|   stm32f768a_778a_769_779_wlcsp180 IBIS Model
[IBIS ver]   4.2
[File name]  stm32f768a_778a_769_779_wlcsp180.ibs
[File Rev]   1.0
[Date]   24-06-2015
[Source] Data Created at STMicroelectronics
[Notes]   File originated from ELDO simulations.
[Disclaimer]  This information is for modeling purpose only and is
   not guaranted. The information is subject to change without
   notice.
[Copyright] Copyright 2016 STMicroelectronics Inc.
[Component] stm32f768a_778a_769_779_wlcsp180
[Manufacturer] STMicroelectronics
[Package]
| variable   typ   min   max
R_pkg   0.0   NA   NA
L_pkg   0.0H   NA   NA
C_pkg   0.0F   NA   NA
[Pin]   signal_name   model_name   R_pin   L_pin   C_pin
E10 PE2 io8p_arsudq_ft
F10 PE3 io8p_arsudq_ft
C12 PE4 io8p_arsudq_ft
D12 PE5 io8p_arsudq_ft
E11 PE6 io8p_arsudq_ft
C13 VBAT POWER
D13 PC13 io8p_arwsudq_ft_v33
E12 PC14-OSC32_IN io8p_arwsudq_ft_v33
E13 PC15-OSC32_OUT io8p_arsudq_ft
G10 PI9 io8p_arsudq_ft
H10 PI10 io8p_arsudq_ft
F11 PI11 io8p_arsudq_ft_v33
F13 VSS GND
F12 VDD POWER
G11 PF0 io8p_arsudq_i2cin_ft
G12 PF1 io8p_arsudq_i2cin_ft
G13 PF2 io8p_arsudq_ft
H11 PF3 io8p_arwsudq_ft
H12 PF4 io8p_arwsudq_ft
H13 PF5 io8p_arwsudq_ft
J13 VSS GND
J12 VDD POWER
K11 PF10 io8p_arwsudq_ft
K12 PH0-OSC_IN io8p_arsudq_ft
K13 PH1-OSC_OUT io8p_arsudq_ft
L11 NRST ioreset_ft_v33
L12 PC0 io8p_ar3wsudq_ft
L13 PC1 io8p_ar3wsudq_ft_v33
M11 VSSA GND
M12 VDDA POWER
M13 PA0-WKUP io8p_ar3wsudq_ft_v33
J11 PA1 io8p_ar3wsudq_ft
J10 PA2 io8p_ar3wsudq_ft_v33
L10 PH2 io8p_arsudq_ft
K10 PH3 io8p_arsudq_ft
N12 PH4 io8p_arsudq_i2cin_ft
N11 PH5 io8p_arsudq_i2cin_ft
M10 PA3 io8p_ar3wsudq_ft
J9 VSS GND
K9 VDD POWER
L9 PA4 io8p_ar3wsudq_ft
Q11 PA5 io8p_ar3wsudq_ft
N10 PA6 io8p_ar3wsudq_ft
M9 PA7 io8p_ar3wsudq_ft
P10 PB0 io8p_ar3wsudq_ft
J8 PB1 io8p_ar3wsudq_ft
J7 PB2 io8p_ar3wsudq_ft
N9 PF11 io8p_arsudq_ft
K7 PF12 io8p_arsudq_ft
Q9 VSS GND
M8 VDD POWER
L8 PF13 io8p_arsudq_ft
K8 PF14 io8p_arsudq_i2cin_ft
Q8 PF15 io8p_arsudq_i2cin_ft
N8 PG0 io8p_arsudq_ft
L7 PG1 io8p_arsudq_ft
M7 PE7 io8p_arsudq_ft
N7 PE8 io8p_arsudq_ft
P7 PE9 io8p_arsudq_ft
J6 PE10 io8p_arsudq_ft
K6 PE11 io8p_arsudq_ft
L6 PE12 io8p_arsudq_ft
P6 PE13 io8p_arsudq_ft
N6 PE14 io8p_arsudq_ft
M6 PE15 io8p_ar3wsudq_ft
K5 PB10 io8p_arsudq_i2cin_ft
L5 PB11 io8p_arsudq_i2cin_ft
P5 VCAP_1 POWER
N5 VSS GND
P4 VDD POWER
M5 PH8 io8p_arsudq_i2cin_ft
K4 PH9 io8p_arsudq_ft
L4 PH10 io8p_arsudq_ft
M4 PH11 io8p_arsudq_i2cin_ft
P3 PH12 io8p_arsudq_i2cin_ft
N4 VSS GND
H8 PB12 io8usb_id_otg_ft
J5 PB13 io8usb_vbus_otg_ft
N3 PB14 io8usb_lsfs_otg_ft
N2 PB15 io8usb_lsfs_otg_ft
M3 PD8 io8p_arsudq_ft
L3 PD9 io8p_arsudq_ft
M2 PD10 io8p_arsudq_ft
K3 PD11 io8p_arsudq_ft
J4 PD12 io8p_arsudq_i2cin_ft
L2 PD13 io8p_arsudq_i2cin_ft
M1 VSS GND
L1 PD14 io8p_arsudq_ft
K2 PD15 io8p_arsudq_ft
K1 VDDDSI POWER
H6 VCAPDSI POWER
J3 VDD12DSI POWER
J1 DSI_D0P NC
J2 DSI_D0N NC
H5 VSSDSI GND
H4 DSI_CKP NC
H3 DSI_CKN NC
H1 DSI_D1P NC
H2 DSI_D1N NC
H9 PG2 io8p_arsudq_ft
G9 PG3 io8p_arsudq_ft
G1 PG4 io8p_arsudq_ft
G2 PG5 io8p_arsudq_ft
G3 PG6 io8p_arsudq_ft
G4 PG7 io8p_arsudq_ft
G5 PG8 io8p_arsudq_ft
F1 VSS GND
F2 VDDUSB POWER
G6 PC6 io8p_arsudq_ft
F3 PC7 io8p_arsudq_ft
G8 PC8 io8p_arsudq_ft
E1 PC9 io8p_arsudq_i2cin_ft
E2 PA8 io8p_arsudq_i2cin_ft
F4 PA9 io8usb_vbus_otg_ft
F5 PA10 io8usb_id_otg_ft
E3 PA11 io8usb_lsfs_otg_ft
D1 PA12 io8usb_lsfs_otg_ft
D2 PA13 io8p_arsudq_ft
C1 VCAP_2 POWER
C2 VSS POWER
B2 VDD POWER
F6 PH13 io8p_arsudq_ft
F7 PH14 io8p_arsudq_ft
E5 PH15 io8p_arsudq_ft
E4 PI0 io8p_arsudq_ft
B3 PI1 io8p_arsudq_ft
C3 PI2 io8p_arsudq_ft
D3 PI3 io8p_arsudq_ft
A3 PA14 io8p_arsudq_ft
F8 PA15 io8p_arsudq_ft
B4 PC10 io8p_arsudq_ft
C4 PC11 io8p_arsudq_ft
D4 PC12 io8p_arsudq_ft
A4 PD0 io8p_arsudq_ft
D5 PD1 io8p_arsudq_ft
D6 PD2 io8p_arsudq_ft
B5 PD3 io8p_arsudq_ft
A5 PD4 io8p_arsudq_ft
C5 PD5 io8p_arsudq_ft
B6 VSS GND
A6 VDDSDMMC POWER
E6 PD6 io8p_arsudq_ft
E7 PD7 io8p_arsudq_ft
C6 PG9 io8p_arsudq_ft
A7 PG10 io8p_arsudq_ft
B7 PG11 io8p_arsudq_ft
D7 PG12 io8p_arsudq_ft
C7 PG13 io8p_arsudq_ft
A8 VSS GND
B8 VDD POWER
F9 PG15 io8p_arsudq_ft
E8 PB3 io8p_arsudq_ft
D8 PB4 io8p_arsudq_ft
A9 PB5 io8p_ar3wsudq_ft
B9 PB6 io8p_arsudq_i2cin_ft
C8 PB7 io8p_arsudq_i2cin_ft
A10 BOOT0 vpp_test_hv
E9 PB8 io8p_arsudq_i2cin_ft
D9 PB9 io8p_arsudq_i2cin_ft
C9 PE0 io8p_arsudq_ft
B10 PE1 io8p_arsudq_ft
A11 VSS GND
C10 PDR_ON NC
B11 VDD POWER
D10 PI4 io8p_arsudq_ft
D11 PI5 io8p_arsudq_ft
C11 PI6 io8p_arsudq_ft
B12 PI7 io8p_arsudq_ft
[Diff Pin]   inv_pin   vdiff   tdelay_typ  tdelay_min  tdelay_max
E3   D1   200mV   NA   NA   NA
N3   N2   200mV   NA   NA   NA
[Model Selector] io8p_ar3wsudq_ft
io8p00_ar3wsudq_ft_pd_lv  "SPEED00 1P8V, PD=40kOhm"
io8p00_ar3wsudq_ft_pu_lv  "SPEED00 1P8V, PU=40kOhm"
io8p00_ar3wsudq_ft_lv  "SPEED00 1P8V"
io8p01_ar3wsudq_ft_pd_lv  "SPEED01 1P8V, PD=40kOhm"
io8p01_ar3wsudq_ft_pu_lv  "SPEED01 1P8V, PU=40kOhm"
io8p01_ar3wsudq_ft_lv  "SPEED01 1P8V"
io8p10_ar3wsudq_ft_pd_lv  "SPEED10 1P8V, PD=40kOhm"
io8p10_ar3wsudq_ft_pu_lv  "SPEED10 1P8V, PU=40kOhm"
io8p10_ar3wsudq_ft_lv  "SPEED10 1P8V"
io8p11_ar3wsudq_ft_pd_lv  "SPEED11 1P8V, PD=40kOhm"
io8p11_ar3wsudq_ft_pu_lv  "SPEED11 1P8V, PU=40kOhm"
io8p11_ar3wsudq_ft_lv  "SPEED11 1P8V"
io8p00_ar3wsudq_ft_pd  "SPEED00, PD=40kOhm"
io8p00_ar3wsudq_ft_pu  "SPEED00, PU=40kOhm"
io8p00_ar3wsudq_ft  "SPEED00"
io8p01_ar3wsudq_ft_pd  "SPEED01, PD=40kOhm"
io8p01_ar3wsudq_ft_pu  "SPEED01, PU=40kOhm"
io8p01_ar3wsudq_ft  "SPEED01"
io8p10_ar3wsudq_ft_pd  "SPEED10, PD=40kOhm"
io8p10_ar3wsudq_ft_pu  "SPEED10, PU=40kOhm"
io8p10_ar3wsudq_ft  "SPEED10"
io8p11_ar3wsudq_ft_pd  "SPEED11, PD=40kOhm"
io8p11_ar3wsudq_ft_pu  "SPEED11, PU=40kOhm"
io8p11_ar3wsudq_ft  "SPEED11"
[Model Selector] io8p_ar3wsudq_ft_v33
io8p00_ar3wsudq_ft_v33_pd_lv  "SPEED00 1P8V, PD=40kOhm"
io8p00_ar3wsudq_ft_v33_pu_lv  "SPEED00 1P8V, PU=40kOhm"
io8p00_ar3wsudq_ft_v33_lv  "SPEED00 1P8V"
io8p01_ar3wsudq_ft_v33_pd_lv  "SPEED01 1P8V, PD=40kOhm"
io8p01_ar3wsudq_ft_v33_pu_lv  "SPEED01 1P8V, PU=40kOhm"
io8p01_ar3wsudq_ft_v33_lv  "SPEED01 1P8V"
io8p10_ar3wsudq_ft_v33_pd_lv  "SPEED10 1P8V, PD=40kOhm"
io8p10_ar3wsudq_ft_v33_pu_lv  "SPEED10 1P8V, PU=40kOhm"
io8p10_ar3wsudq_ft_v33_lv  "SPEED10 1P8V"
io8p11_ar3wsudq_ft_v33_pd_lv  "SPEED11 1P8V, PD=40kOhm"
io8p11_ar3wsudq_ft_v33_pu_lv  "SPEED11 1P8V, PU=40kOhm"
io8p11_ar3wsudq_ft_v33_lv  "SPEED11 1P8V"
io8p00_ar3wsudq_ft_v33_pd  "SPEED00, PD=40kOhm"
io8p00_ar3wsudq_ft_v33_pu  "SPEED00, PU=40kOhm"
io8p00_ar3wsudq_ft_v33  "SPEED00"
io8p01_ar3wsudq_ft_v33_pd  "SPEED01, PD=40kOhm"
io8p01_ar3wsudq_ft_v33_pu  "SPEED01, PU=40kOhm"
io8p01_ar3wsudq_ft_v33  "SPEED01"
io8p10_ar3wsudq_ft_v33_pd  "SPEED10, PD=40kOhm"
io8p10_ar3wsudq_ft_v33_pu  "SPEED10, PU=40kOhm"
io8p10_ar3wsudq_ft_v33  "SPEED10"
io8p11_ar3wsudq_ft_v33_pd  "SPEED11, PD=40kOhm"
io8p11_ar3wsudq_ft_v33_pu  "SPEED11, PU=40kOhm"
io8p11_ar3wsudq_ft_v33  "SPEED11"
[Model Selector] io8p_arsudq_ft
io8p00_arsudq_ft_pd_lv  "SPEED00 1P8V, PD=40kOhm"
io8p00_arsudq_ft_pu_lv  "SPEED00 1P8V, PU=40kOhm"
io8p00_arsudq_ft_lv  "SPEED00 1P8V"
io8p01_arsudq_ft_pd_lv  "SPEED01 1P8V, PD=40kOhm"
io8p01_arsudq_ft_pu_lv  "SPEED01 1P8V, PU=40kOhm"
io8p01_arsudq_ft_lv  "SPEED01 1P8V"
io8p10_arsudq_ft_pd_lv  "SPEED10 1P8V, PD=40kOhm"
io8p10_arsudq_ft_pu_lv  "SPEED10 1P8V, PU=40kOhm"
io8p10_arsudq_ft_lv  "SPEED10 1P8V"
io8p11_arsudq_ft_pd_lv  "SPEED11 1P8V, PD=40kOhm"
io8p11_arsudq_ft_pu_lv  "SPEED11 1P8V, PU=40kOhm"
io8p11_arsudq_ft_lv  "SPEED11 1P8V"
io8p00_arsudq_ft_pd  "SPEED00, PD=40kOhm"
io8p00_arsudq_ft_pu  "SPEED00, PU=40kOhm"
io8p00_arsudq_ft  "SPEED00"
io8p01_arsudq_ft_pd  "SPEED01, PD=40kOhm"
io8p01_arsudq_ft_pu  "SPEED01, PU=40kOhm"
io8p01_arsudq_ft  "SPEED01"
io8p10_arsudq_ft_pd  "SPEED10, PD=40kOhm"
io8p10_arsudq_ft_pu  "SPEED10, PU=40kOhm"
io8p10_arsudq_ft  "SPEED10"
io8p11_arsudq_ft_pd  "SPEED11, PD=40kOhm"
io8p11_arsudq_ft_pu  "SPEED11, PU=40kOhm"
io8p11_arsudq_ft  "SPEED11"
[Model Selector] io8p_arsudq_i2cin_ft
io8p00_arsudq_i2cin_ft_pd_lv  "SPEED00 1P8V, PD=40kOhm"
io8p00_arsudq_i2cin_ft_pu_lv  "SPEED00 1P8V, PU=40kOhm"
io8p00_arsudq_i2cin_ft_lv  "SPEED00 1P8V"
io8p01_arsudq_i2cin_ft_pd_lv  "SPEED01 1P8V, PD=40kOhm"
io8p01_arsudq_i2cin_ft_pu_lv  "SPEED01 1P8V, PU=40kOhm"
io8p01_arsudq_i2cin_ft_lv  "SPEED01 1P8V"
io8p10_arsudq_i2cin_ft_pd_lv  "SPEED10 1P8V, PD=40kOhm"
io8p10_arsudq_i2cin_ft_pu_lv  "SPEED10 1P8V, PU=40kOhm"
io8p10_arsudq_i2cin_ft_lv  "SPEED10 1P8V"
io8p11_arsudq_i2cin_ft_pd_lv  "SPEED11 1P8V, PD=40kOhm"
io8p11_arsudq_i2cin_ft_pu_lv  "SPEED11 1P8V, PU=40kOhm"
io8p11_arsudq_i2cin_ft_lv  "SPEED11 1P8V"
io8p00_arsudq_i2cin_ft_pd  "SPEED00, PD=40kOhm"
io8p00_arsudq_i2cin_ft_pu  "SPEED00, PU=40kOhm"
io8p00_arsudq_i2cin_ft  "SPEED00"
io8p01_arsudq_i2cin_ft_pd  "SPEED01, PD=40kOhm"
io8p01_arsudq_i2cin_ft_pu  "SPEED01, PU=40kOhm"
io8p01_arsudq_i2cin_ft  "SPEED01"
io8p10_arsudq_i2cin_ft_pd  "SPEED10, PD=40kOhm"
io8p10_arsudq_i2cin_ft_pu  "SPEED10, PU=40kOhm"
io8p10_arsudq_i2cin_ft  "SPEED10"
io8p11_arsudq_i2cin_ft_pd  "SPEED11, PD=40kOhm"
io8p11_arsudq_i2cin_ft_pu  "SPEED11, PU=40kOhm"
io8p11_arsudq_i2cin_ft  "SPEED11"
[Model Selector] io8p_arwsudq_ft_v33
io8p00_arwsudq_ft_v33_pd_lv  "SPEED00 1P8V, PD=40kOhm"
io8p00_arwsudq_ft_v33_pu_lv  "SPEED00 1P8V, PU=40kOhm"
io8p00_arwsudq_ft_v33_lv  "SPEED00 1P8V"
io8p01_arwsudq_ft_v33_pd_lv  "SPEED01 1P8V, PD=40kOhm"
io8p01_arwsudq_ft_v33_pu_lv  "SPEED01 1P8V, PU=40kOhm"
io8p01_arwsudq_ft_v33_lv  "SPEED01 1P8V"
io8p10_arwsudq_ft_v33_pd_lv  "SPEED10 1P8V, PD=40kOhm"
io8p10_arwsudq_ft_v33_pu_lv  "SPEED10 1P8V, PU=40kOhm"
io8p10_arwsudq_ft_v33_lv  "SPEED10 1P8V"
io8p11_arwsudq_ft_v33_pd_lv  "SPEED11 1P8V, PD=40kOhm"
io8p11_arwsudq_ft_v33_pu_lv  "SPEED11 1P8V, PU=40kOhm"
io8p11_arwsudq_ft_v33_lv  "SPEED11 1P8V"
io8p00_arwsudq_ft_v33_pd  "SPEED00, PD=40kOhm"
io8p00_arwsudq_ft_v33_pu  "SPEED00, PU=40kOhm"
io8p00_arwsudq_ft_v33  "SPEED00"
io8p01_arwsudq_ft_v33_pd  "SPEED01, PD=40kOhm"
io8p01_arwsudq_ft_v33_pu  "SPEED01, PU=40kOhm"
io8p01_arwsudq_ft_v33  "SPEED01"
io8p10_arwsudq_ft_v33_pd  "SPEED10, PD=40kOhm"
io8p10_arwsudq_ft_v33_pu  "SPEED10, PU=40kOhm"
io8p10_arwsudq_ft_v33  "SPEED10"
io8p11_arwsudq_ft_v33_pd  "SPEED11, PD=40kOhm"
io8p11_arwsudq_ft_v33_pu  "SPEED11, PU=40kOhm"
io8p11_arwsudq_ft_v33  "SPEED11"
[Model Selector] io8usb_id_otg_ft
io8p00_id_otg_ft_pd_lv  "SPEED00 1P8V, PD=14kOhm"
io8p00_id_otg_ft_pu_lv  "SPEED00 1P8V, PU=14kOhm"
io8p00_id_otg_ft_lv  "SPEED00 1P8V"
io8p01_id_otg_ft_pd_lv  "SPEED01 1P8V, PD=14kOhm"
io8p01_id_otg_ft_pu_lv  "SPEED01 1P8V, PU=14kOhm"
io8p01_id_otg_ft_lv  "SPEED01 1P8V"
io8p10_id_otg_ft_pd_lv  "SPEED10 1P8V, PD=14kOhm"
io8p10_id_otg_ft_pu_lv  "SPEED10 1P8V, PU=14kOhm"
io8p10_id_otg_ft_lv  "SPEED10 1P8V"
io8p11_id_otg_ft_pd_lv  "SPEED11 1P8V, PD=14kOhm"
io8p11_id_otg_ft_pu_lv  "SPEED11 1P8V, PU=14kOhm"
io8p11_id_otg_ft_lv  "SPEED11 1P8V"
io8p00_id_otg_ft_pd  "SPEED00, PD=14kOhm"
io8p00_id_otg_ft_pu  "SPEED00, PU=14kOhm"
io8p00_id_otg_ft  "SPEED00"
io8p01_id_otg_ft_pd  "SPEED01, PD=14kOhm"
io8p01_id_otg_ft_pu  "SPEED01, PU=14kOhm"
io8p01_id_otg_ft  "SPEED01"
io8p10_id_otg_ft_pd  "SPEED10, PD=14kOhm"
io8p10_id_otg_ft_pu  "SPEED10, PU=14kOhm"
io8p10_id_otg_ft  "SPEED10"
io8p11_id_otg_ft_pd  "SPEED11, PD=14kOhm"
io8p11_id_otg_ft_pu  "SPEED11, PU=14kOhm"
io8p11_id_otg_ft  "SPEED11"
[Model Selector] io8usb_lsfs_otg_ft
io8usb_ls_otg_ft_dpdn_pd  "LS USB DP/DN IO + PD=20kOhm"
io8usb_ls_otg_ft_dpdn_pupu2  "LS USB DP/DN IO + PU/PU2=2.2kOhm"
io8usb_ls_otg_ft_dpdn_pu2  "LS USB DP/DN IO + PU2=1.2kOhm"
io8usb_ls_otg_ft_dpdn_pu  "LS USB DP/DN IO + PU=1.2kOhm"
io8usb_ls_otg_ft_dpdn  "LS USB DP/DN IO"
io8usb_fs_otg_ft_dpdn_pd  "HS USB DP/DN IO + PD=20kOhm"
io8usb_fs_otg_ft_dpdn_pupu2  "HS USB DP/DN IO + PU/PU2=2.2kOhm"
io8usb_fs_otg_ft_dpdn_pu2  "HS USB DP/DN IO + PU2=1.2kOhm"
io8usb_fs_otg_ft_dpdn_pu  "HS USB DP/DN IO + PU=1.2kOhm"
io8usb_fs_otg_ft_dpdn  "HS USB DP/DN IO"
io8p00_lsfs_otg_ft_pd_lv  "SPEED00 1P8V, PD=40kOhm"
io8p00_lsfs_otg_ft_pu_lv  "SPEED00 1P8V, PU=40kOhm"
io8p00_lsfs_otg_ft_lv  "SPEED00 1P8V"
io8p01_lsfs_otg_ft_pd_lv  "SPEED01 1P8V, PD=40kOhm"
io8p01_lsfs_otg_ft_pu_lv  "SPEED01 1P8V, PU=40kOhm"
io8p01_lsfs_otg_ft_lv  "SPEED01 1P8V"
io8p10_lsfs_otg_ft_pd_lv  "SPEED10 1P8V, PD=40kOhm"
io8p10_lsfs_otg_ft_pu_lv  "SPEED10 1P8V, PU=40kOhm"
io8p10_lsfs_otg_ft_lv  "SPEED10 1P8V"
io8p11_lsfs_otg_ft_pd_lv  "SPEED11 1P8V, PD=40kOhm"
io8p11_lsfs_otg_ft_pu_lv  "SPEED11 1P8V, PU=40kOhm"
io8p11_lsfs_otg_ft_lv  "SPEED11 1P8V"
io8p00_lsfs_otg_ft_pd  "SPEED00, PD=40kOhm"
io8p00_lsfs_otg_ft_pu  "SPEED00, PU=40kOhm"
io8p00_lsfs_otg_ft  "SPEED00"
io8p01_lsfs_otg_ft_pd  "SPEED01, PD=40kOhm"
io8p01_lsfs_otg_ft_pu  "SPEED01, PU=40kOhm"
io8p01_lsfs_otg_ft  "SPEED01"
io8p10_lsfs_otg_ft_pd  "SPEED10, PD=40kOhm"
io8p10_lsfs_otg_ft_pu  "SPEED10, PU=40kOhm"
io8p10_lsfs_otg_ft  "SPEED10"
io8p11_lsfs_otg_ft_pd  "SPEED11, PD=40kOhm"
io8p11_lsfs_otg_ft_pu  "SPEED11, PU=40kOhm"
io8p11_lsfs_otg_ft  "SPEED11"
[Model Selector] io8usb_vbus_otg_ft
io8psenb_vbus_otg_ft  "VBUS PULSE, SENSE VB"
io8psenab_vbus_otg_ft  "VBUS PULSE, SENSE VA and VB"
io8psena_vbus_otg_ft  "VBUS PULSE, SENSE VA"
io8psen_vbus_otg_ft  "VBUS PULSE"
io8p00_vbus_otg_ft_pd_lv  "SPEED00 1P8V, PD=40kOhm"
io8p00_vbus_otg_ft_pu_lv  "SPEED00 1P8V, PU=40kOhm"
io8p00_vbus_otg_ft_lv  "SPEED00 1P8V"
io8p01_vbus_otg_ft_pd_lv  "SPEED01 1P8V, PD=40kOhm"
io8p01_vbus_otg_ft_pu_lv  "SPEED01 1P8V, PU=40kOhm"
io8p01_vbus_otg_ft_lv  "SPEED01 1P8V"
io8p10_vbus_otg_ft_pd_lv  "SPEED10 1P8V, PD=40kOhm"
io8p10_vbus_otg_ft_pu_lv  "SPEED10 1P8V, PU=40kOhm"
io8p10_vbus_otg_ft_lv  "SPEED10 1P8V"
io8p11_vbus_otg_ft_pd_lv  "SPEED11 1P8V, PD=40kOhm"
io8p11_vbus_otg_ft_pu_lv  "SPEED11 1P8V, PU=40kOhm"
io8p11_vbus_otg_ft_lv  "SPEED11 1P8V"
io8p00_vbus_otg_ft_pd  "SPEED00, PD=40kOhm"
io8p00_vbus_otg_ft_pu  "SPEED00, PU=40kOhm"
io8p00_vbus_otg_ft  "SPEED00"
io8p01_vbus_otg_ft_pd  "SPEED01, PD=40kOhm"
io8p01_vbus_otg_ft_pu  "SPEED01, PU=40kOhm"
io8p01_vbus_otg_ft  "SPEED01"
io8p10_vbus_otg_ft_pd  "SPEED10, PD=40kOhm"
io8p10_vbus_otg_ft_pu  "SPEED10, PU=40kOhm"
io8p10_vbus_otg_ft  "SPEED10"
io8p11_vbus_otg_ft_pd  "SPEED11, PD=40kOhm"
io8p11_vbus_otg_ft_pu  "SPEED11, PU=40kOhm"
io8p11_vbus_otg_ft  "SPEED11"
[Model Selector] ioreset_ft_v33
ioreset_ft_v33_pu_lv  "ioreset 1P8V + PU=40kOhm"
ioreset_ft_v33_nopu_lv  "ioreset 1P8V"
ioreset_ft_v33_pu  "ioreset + PU=40kOhm"
ioreset_ft_v33_nopu  "ioreset"
[Model Selector] vpp_test_hv
vpp_test_hv_2p4  "Input Buffer 1P8V"
vpp_test_hv_3p3  "Input Buffer"
[Model Selector] io8p_arwsudq_ft
io8p00_arwsudq_ft_pd_lv  "SPEED00 1P8V, PD=40kOhm"
io8p00_arwsudq_ft_pu_lv  "SPEED00 1P8V, PU=40kOhm"
io8p00_arwsudq_ft_lv  "SPEED00 1P8V"
io8p01_arwsudq_ft_pd_lv  "SPEED01 1P8V, PD=40kOhm"
io8p01_arwsudq_ft_pu_lv  "SPEED01 1P8V, PU=40kOhm"
io8p01_arwsudq_ft_lv  "SPEED01 1P8V"
io8p10_arwsudq_ft_pd_lv  "SPEED10 1P8V, PD=40kOhm"
io8p10_arwsudq_ft_pu_lv  "SPEED10 1P8V, PU=40kOhm"
io8p10_arwsudq_ft_lv  "SPEED10 1P8V"
io8p11_arwsudq_ft_pd_lv  "SPEED11 1P8V, PD=40kOhm"
io8p11_arwsudq_ft_pu_lv  "SPEED11 1P8V, PU=40kOhm"
io8p11_arwsudq_ft_lv  "SPEED11 1P8V"
io8p00_arwsudq_ft_pd  "SPEED00, PD=40kOhm"
io8p00_arwsudq_ft_pu  "SPEED00, PU=40kOhm"
io8p00_arwsudq_ft  "SPEED00"
io8p01_arwsudq_ft_pd  "SPEED01, PD=40kOhm"
io8p01_arwsudq_ft_pu  "SPEED01, PU=40kOhm"
io8p01_arwsudq_ft  "SPEED01"
io8p10_arwsudq_ft_pd  "SPEED10, PD=40kOhm"
io8p10_arwsudq_ft_pu  "SPEED10, PU=40kOhm"
io8p10_arwsudq_ft  "SPEED10"
io8p11_arwsudq_ft_pd  "SPEED11, PD=40kOhm"
io8p11_arwsudq_ft_pu  "SPEED11, PU=40kOhm"
io8p11_arwsudq_ft  "SPEED11"
[Model Selector] io8p_arsudq_ft_v33
io8p00_arsudq_ft_v33_pd_lv  "SPEED00 1P8V, PD=40kOhm"
io8p00_arsudq_ft_v33_pu_lv  "SPEED00 1P8V, PU=40kOhm"
io8p00_arsudq_ft_v33_lv  "SPEED00 1P8V"
io8p01_arsudq_ft_v33_pd_lv  "SPEED01 1P8V, PD=40kOhm"
io8p01_arsudq_ft_v33_pu_lv  "SPEED01 1P8V, PU=40kOhm"
io8p01_arsudq_ft_v33_lv  "SPEED01 1P8V"
io8p10_arsudq_ft_v33_pd_lv  "SPEED10 1P8V, PD=40kOhm"
io8p10_arsudq_ft_v33_pu_lv  "SPEED10 1P8V, PU=40kOhm"
io8p10_arsudq_ft_v33_lv  "SPEED10 1P8V"
io8p11_arsudq_ft_v33_pd_lv  "SPEED11 1P8V, PD=40kOhm"
io8p11_arsudq_ft_v33_pu_lv  "SPEED11 1P8V, PU=40kOhm"
io8p11_arsudq_ft_v33_lv  "SPEED11 1P8V"
io8p00_arsudq_ft_v33_pd  "SPEED00, PD=40kOhm"
io8p00_arsudq_ft_v33_pu  "SPEED00, PU=40kOhm"
io8p00_arsudq_ft_v33  "SPEED00"
io8p01_arsudq_ft_v33_pd  "SPEED01, PD=40kOhm"
io8p01_arsudq_ft_v33_pu  "SPEED01, PU=40kOhm"
io8p01_arsudq_ft_v33  "SPEED01"
io8p10_arsudq_ft_v33_pd  "SPEED10, PD=40kOhm"
io8p10_arsudq_ft_v33_pu  "SPEED10, PU=40kOhm"
io8p10_arsudq_ft_v33  "SPEED10"
io8p11_arsudq_ft_v33_pd  "SPEED11, PD=40kOhm"
io8p11_arsudq_ft_v33_pu  "SPEED11, PU=40kOhm"
io8p11_arsudq_ft_v33  "SPEED11"
| Models and submodels in the file (260): io8p00_ar3wsudq_ft_pd_lv (I/O), io8p00_ar3wsudq_ft_pu_lv (I/O), io8p00_ar3wsudq_ft_lv (I/O), io8p01_ar3wsudq_ft_pd_lv (I/O), io8p01_ar3wsudq_ft_pu_lv (I/O), io8p01_ar3wsudq_ft_lv (I/O), io8p10_ar3wsudq_ft_pd_lv (I/O), io8p10_ar3wsudq_ft_pu_lv (I/O), io8p10_ar3wsudq_ft_lv (I/O), io8p11_ar3wsudq_ft_pd_lv (I/O), io8p11_ar3wsudq_ft_pu_lv (I/O), io8p11_ar3wsudq_ft_lv (I/O), io8p00_ar3wsudq_ft_pd (I/O), io8p00_ar3wsudq_ft_pu (I/O), io8p00_ar3wsudq_ft (I/O), io8p01_ar3wsudq_ft_pd (I/O), io8p01_ar3wsudq_ft_pu (I/O), io8p01_ar3wsudq_ft (I/O), io8p10_ar3wsudq_ft_pd (I/O), io8p10_ar3wsudq_ft_pu (I/O), io8p10_ar3wsudq_ft (I/O), io8p11_ar3wsudq_ft_pd (I/O), io8p11_ar3wsudq_ft_pu (I/O), io8p11_ar3wsudq_ft (I/O), io8p00_ar3wsudq_ft_v33_pd_lv (I/O), io8p00_ar3wsudq_ft_v33_pu_lv (I/O), io8p00_ar3wsudq_ft_v33_lv (I/O), io8p01_ar3wsudq_ft_v33_pd_lv (I/O), io8p01_ar3wsudq_ft_v33_pu_lv (I/O), io8p01_ar3wsudq_ft_v33_lv (I/O), io8p10_ar3wsudq_ft_v33_pd_lv (I/O), io8p10_ar3wsudq_ft_v33_pu_lv (I/O), io8p10_ar3wsudq_ft_v33_lv (I/O), io8p11_ar3wsudq_ft_v33_pd_lv (I/O), io8p11_ar3wsudq_ft_v33_pu_lv (I/O), io8p11_ar3wsudq_ft_v33_lv (I/O), io8p00_ar3wsudq_ft_v33_pd (I/O), io8p00_ar3wsudq_ft_v33_pu (I/O), io8p00_ar3wsudq_ft_v33 (I/O), io8p01_ar3wsudq_ft_v33_pd (I/O), io8p01_ar3wsudq_ft_v33_pu (I/O), io8p01_ar3wsudq_ft_v33 (I/O), io8p10_ar3wsudq_ft_v33_pd (I/O), io8p10_ar3wsudq_ft_v33_pu (I/O), io8p10_ar3wsudq_ft_v33 (I/O), io8p11_ar3wsudq_ft_v33_pd (I/O), io8p11_ar3wsudq_ft_v33_pu (I/O), io8p11_ar3wsudq_ft_v33 (I/O), io8p00_arsudq_ft_pd_lv (I/O), io8p00_arsudq_ft_pu_lv (I/O), io8p00_arsudq_ft_lv (I/O), io8p01_arsudq_ft_pd_lv (I/O), io8p01_arsudq_ft_pu_lv (I/O), io8p01_arsudq_ft_lv (I/O), io8p10_arsudq_ft_pd_lv (I/O), io8p10_arsudq_ft_pu_lv (I/O), io8p10_arsudq_ft_lv (I/O), io8p11_arsudq_ft_pd_lv (I/O), io8p11_arsudq_ft_pu_lv (I/O), io8p11_arsudq_ft_lv (I/O), io8p00_arsudq_ft_pd (I/O), io8p00_arsudq_ft_pu (I/O), io8p00_arsudq_ft (I/O), io8p01_arsudq_ft_pd (I/O), io8p01_arsudq_ft_pu (I/O), io8p01_arsudq_ft (I/O), io8p10_arsudq_ft_pd (I/O), io8p10_arsudq_ft_pu (I/O), io8p10_arsudq_ft (I/O), io8p11_arsudq_ft_pd (I/O), io8p11_arsudq_ft_pu (I/O), io8p11_arsudq_ft (I/O), io8p00_arsudq_i2cin_ft_pd_lv (I/O), io8p00_arsudq_i2cin_ft_pu_lv (I/O), io8p00_arsudq_i2cin_ft_lv (I/O), io8p01_arsudq_i2cin_ft_pd_lv (I/O), io8p01_arsudq_i2cin_ft_pu_lv (I/O), io8p01_arsudq_i2cin_ft_lv (I/O), io8p10_arsudq_i2cin_ft_pd_lv (I/O), io8p10_arsudq_i2cin_ft_pu_lv (I/O)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
